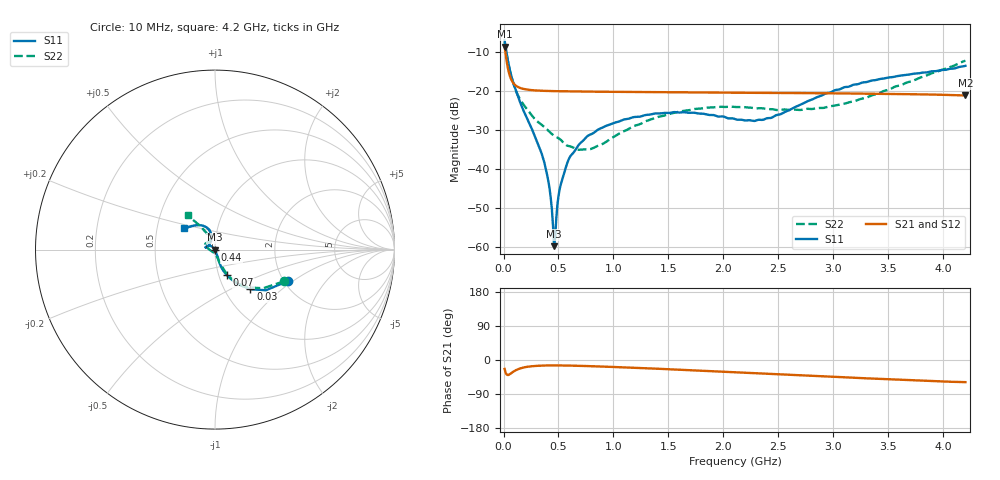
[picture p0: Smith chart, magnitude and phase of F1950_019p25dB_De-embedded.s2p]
! Integrated Device Technology
! Corporate Headquarters
! 6024 Silver Creek Valley Road
! San Jose, CA 95138  USA
! Phone:  1-408-284-8200
! Toll Free:  1-800-223-1366
! Webpage:  http://www.idt.com/
! Timing and RF Division
! 515 Groton Road, Suite 102
! Westford, MA 01886-6024
! Device:  F1950
! Description: 7-bit 0.25 dB Digital Step Attenuator
! Frequency:  150.0 -  4000.00 MHz
! Package:  4x4 mm Thin QFN Plastic Package: 24 pin
! Ports:  2 RF, 12 DC
!  Pin  1  = D0
!  Pin  2  = VDD
!  Pin  3  = Vmode
!  Pin  4  = GND
!  Pin  5  = RF1  =  Port 1
!  Pin  6  = GND
!  Pin  7  = GND
!  Pin  8  = GND
!  Pin  9  = GND
!  Pin 10  = GND
!  Pin 11  = GND
!  Pin 12  = GND
!  Pin 13  = GND
!  Pin 14  = RF2  =  Port 2
!  Pin 15  = GND
!  Pin 16  = LE
!  Pin 17  = CLK
!  Pin 18  = DATE
!  Pin 19  = D6
!  Pin 20  = D5
!  Pin 21  = D4
!  Pin 22  = D3
!  Pin 23  = D2
!  Pin 24  = D1
! State:  77
! Atten State:  19.25 dB
! Voltage:  +5.00 Volts
! Current:  Not Measured mA
! Data:  The device was measured on a the F195X evaluation board which has
!  individual transmission lines to the RF pins.  Data was collected
!  using a calibrated network analyzer.  The evaluation board was
!  de-embedded using a TRL calibration technique.
!  The reference plane is the edge of the package pin.
! Misc:  Board 2019
!  Action Tracker AT0250
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# GHz S dB R 50
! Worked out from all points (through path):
!   420 points, 10 MHz to 4.2 GHz, reference 50 ohm
!   highest |S21| = -8.65 dB at 10 MHz (marker M1); lowest = -21.1 dB at 4.2 GHz (marker M2)
!   group delay of S21, straight-line fit = 30.5 ps
!   lowest |S11| = -59.7 dB at 460 MHz (marker M3), VSWR 1.00, Z = 49.9 - j0.0738 ohm
!   |S11| at or under -10 dB: 26.82 MHz to end of sweep
!   |S22| runs from -35.0 to -7.5 dB; largest |S21 - S12| = 0.00016
!   S11 on the Smith chart (normalised r, x): 10 MHz: 2.11, -0.91; 30 MHz: 1.32, -0.64; 70 MHz: 1.09, -0.32; 440 MHz: 1.00, -0.01; 4.2 GHz: 0.69, +0.17
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0.01  -7.06 -23.1  -8.65 -23.5  -8.65 -23.5  -7.46 -24.6
0.03  -10.57 -48.2  -12.60 -38.8  -12.60 -38.8  -10.94 -48.1
0.07  -16.06 -65.1  -17.04 -34.8  -17.03 -34.8  -16.14 -63.6
0.16  -23.52 -71.5  -19.30 -21.5  -19.29 -21.5  -22.56 -71.0
0.36  -37.22 -67.0  -19.94 -14.7  -19.94 -14.7  -28.95 -77.9
0.41  -43.43 -71.8  -19.99 -14.4  -19.99 -14.4  -30.22 -79.1
0.44  -50.30 -82.6  -20.01 -14.3  -20.01 -14.3  -31.01 -82.2
0.46  -59.71 -134.4  -20.02 -14.3  -20.03 -14.3  -31.43 -84.9
0.48  -52.55 145.1  -20.04 -14.3  -20.04 -14.3  -31.75 -87.4
0.51  -45.21 136.4  -20.05 -14.3  -20.05 -14.4  -32.26 -89.5
0.57  -39.26 132.4  -20.08 -14.6  -20.08 -14.6  -33.83 -97.5
0.61  -36.60 134.6  -20.10 -14.8  -20.10 -14.8  -34.19 -105.0
0.71  -33.06 136.5  -20.13 -15.5  -20.13 -15.6  -34.98 -123.4
0.81  -30.88 139.8  -20.16 -16.4  -20.16 -16.5  -34.66 -144.2
0.99  -28.31 146.6  -20.22 -18.3  -20.22 -18.3  -31.97 -170.3
1.41  -25.74 162.6  -20.31 -23.2  -20.31 -23.2  -26.59 166.3
1.73  -25.54 168.1  -20.37 -27.1  -20.37 -27.1  -24.64 157.4
2.11  -27.23 157.4  -20.44 -32.3  -20.43 -32.3  -24.10 148.0
2.43  -26.89 125.2  -20.49 -36.4  -20.49 -36.4  -24.63 138.0
2.81  -22.12 104.5  -20.55 -41.7  -20.55 -41.7  -24.59 123.0
3.51  -16.51 116.9  -20.73 -51.0  -20.73 -51.1  -19.59 117.5
4.2  -13.55 145.7  -21.14 -58.4  -21.13 -58.5  -12.23 128.7
